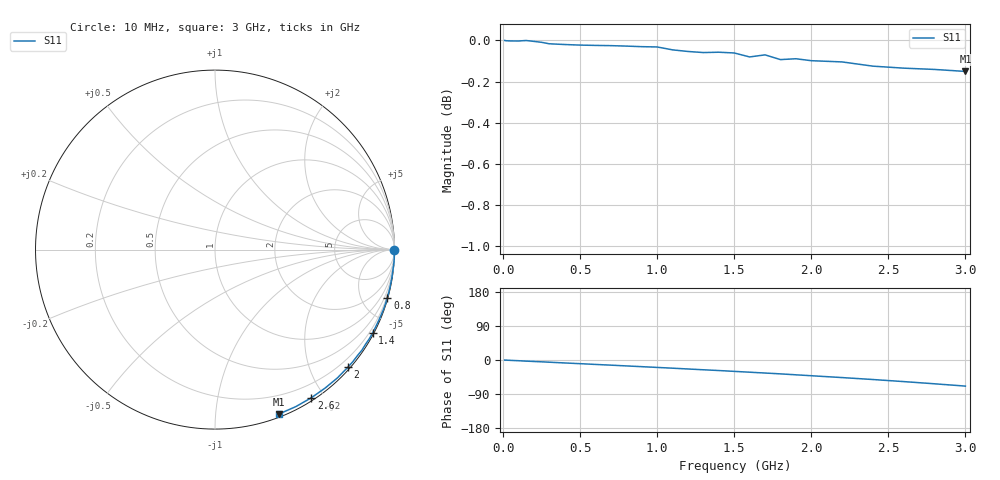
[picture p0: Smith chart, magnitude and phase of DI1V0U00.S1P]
! SIEMENS Small Signal Semiconductors
! BAV99
! Silicon Switching Diode in SOT23
! VR = 1 V
! S-Parameters:  May  1995
# GHz  S  MA  R  50
!  f  S11
! GHz  MAG  ANG
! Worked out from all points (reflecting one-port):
!   30 points, 10 MHz to 3 GHz, reference 50 ohm
!   lowest |S11| = -0.2 dB at 3 GHz (marker M1), VSWR 115.28, Z = 1.36 - j72.9 ohm
!   phase of S11 starts at -0 deg and turns -69 deg over the sweep
!   S11 on the Smith chart (normalised r, x): 10 MHz: open; 800 MHz: 0.09, -7.30; 1.4 GHz: 0.06, -4.04; 2 GHz: 0.05, -2.64; 2.6 GHz: 0.03, -1.84; 3 GHz: 0.03, -1.46
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0.01  1 -0.2
0.05  0.9997 -1.0
0.1  0.9997 -1.9
0.15  1 -3.0
0.2  0.9995 -3.9
0.25  0.999 -4.8
0.4  0.9977 -7.8
0.5  0.9974 -9.7
0.6  0.9972 -11.7
0.7  0.9971 -13.6
0.8  0.9968 -15.6
0.9  0.9965 -17.6
1  0.9964 -19.6
1.1  0.9947 -21.6
1.2  0.9938 -23.7
1.3  0.9932 -25.8
1.4  0.9934 -27.8
1.5  0.993 -30.0
1.6  0.9908 -32.2
1.7  0.992 -34.4
1.8  0.9893 -36.6
1.9  0.9898 -39.1
2  0.9887 -41.5
2.2  0.988 -46.4
2.4  0.9857 -51.5
2.6  0.9846 -57.0
2.8  0.9839 -62.8
3  0.9828 -68.9
